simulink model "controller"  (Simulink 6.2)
settings: Solver=ode45  StartTime=0.0  StopTime=10.0  RelTol=1e-3
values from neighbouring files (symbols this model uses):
  calfa = cos(alfa0*d2r)    [run.m]
  d2r = pi/180    (= 0.0174532925199)    [run.m]
  Kfilt = (wd1^2*wd2^2*wd3^2*wd4^2*wd5^2*wd6^2)/(wn1^2*wn2^2*wn3^2*wn4^2*wn5^2*wn6^2)    (= 0.818930549142)    [run.m]
  klr = lqr(Ap4,Bp4,Q,R)    [run.m]
  kls = lqr(Ap3,Bp3,Q,R)    [run.m]
  salfa = sin(alfa0*d2r)    [run.m]
  Thet0 = 40    [run.m]
  V0 = 18640    [run.m]
  wd1 = 29    [run.m]
  wd2 = 37    [run.m]
  wd3 = 40    [run.m]
  wd4 = 48    [run.m]
  wd5 = 63    [run.m]
  wd6 = 68    [run.m]
  wd7 = 34    [run.m]
  wd8 = 19.1    [run.m]
  wlp = 6.6    [run.m]
  wlp2 = 12    [run.m]
  wlpr = 12    [run.m]
  wn1 = 30    [run.m]
  wn2 = 37.9    [run.m]
  wn3 = 40.2    [run.m]
  wn4 = 48.6    [run.m]
  wn5 = 64    [run.m]
  wn6 = 68.6    [run.m]
  wn7 = 34    [run.m]
  wn8 = 19.1    [run.m]
  zd1 = 0.12    [run.m]
  zd2 = 0.12    [run.m]
  zd3 = 0.1    [run.m]
  zd4 = 0.1    [run.m]
  zd5 = 0.1    [run.m]
  zd6 = 0.1    [run.m]
  zd7 = 0.1    [run.m]
  zd8 = 0.1    [run.m]
  zlp = 0.9    [run.m]
  zlp2 = 0.7    [run.m]
  zlpr = 0.7    [run.m]
  zn1 = 0.008    [run.m]
  zn2 = 0.01    [run.m]
  zn3 = 0.01    [run.m]
  zn4 = 0.02    [run.m]
  zn5 = 0.01    [run.m]
  zn6 = 0.01    [run.m]
  zn7 = 0.01    [run.m]
  zn8 = 0.01    [run.m]

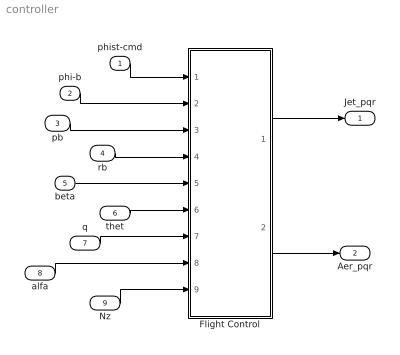
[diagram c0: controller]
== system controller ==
  phist-cmd : Inport  Port=1  LatchInput=off
  phi-b : Inport  Port=2  LatchInput=off
  pb : Inport  Port=3  LatchInput=off
  rb : Inport  Port=4  LatchInput=off
  beta : Inport  Port=5  LatchInput=off
  thet : Inport  Port=6  LatchInput=off
  q : Inport  Port=7  LatchInput=off
  alfa : Inport  Port=8  LatchInput=off
  Nz : Inport  Port=9  LatchInput=off
  Flight Control : Subsystem
  Jet_pqr : Outport
  Aer_pqr : Outport  Port=2
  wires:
  Flight Control/1(Jet_pqr) -> Jet_pqr/1
  Flight Control/2(Aer_pqr) -> Aer_pqr/1
  phi-b/1 -> Flight Control/2(phi)
  pb/1 -> Flight Control/3(pb)
  rb/1 -> Flight Control/4(rb)
  beta/1 -> Flight Control/5(beta)
  thet/1 -> Flight Control/6(thet)
  q/1 -> Flight Control/7(q)
  alfa/1 -> Flight Control/8(alfa)
  Nz/1 -> Flight Control/9(Nz)
  phist-cmd/1 -> Flight Control/1(phis-cmd)

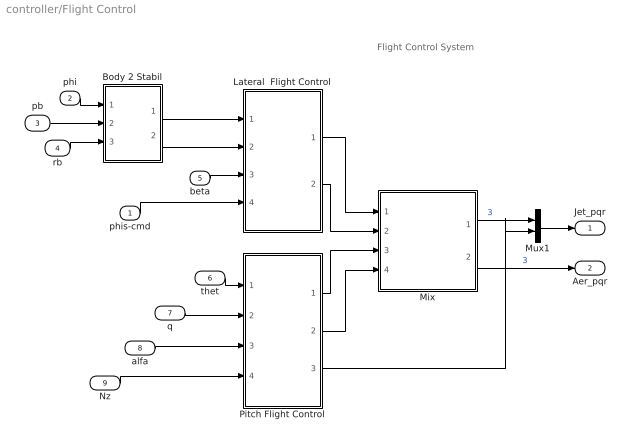
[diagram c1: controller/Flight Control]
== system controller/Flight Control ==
  note: Flight Control System
  phis-cmd : Inport  Port=1  LatchInput=off
  phi : Inport  Port=2  LatchInput=off
  pb : Inport  Port=3  LatchInput=off
  rb : Inport  Port=4  LatchInput=off
  beta : Inport  Port=5  LatchInput=off
  thet : Inport  Port=6  LatchInput=off
  q : Inport  Port=7  LatchInput=off
  alfa : Inport  Port=8  LatchInput=off
  Nz : Inport  Port=9  LatchInput=off
  Body 2 Stabil : Subsystem
  Lateral  Flight Control : Subsystem
  Mix : Subsystem
  Mux1 : Mux  Inputs=[3,1]
  Pitch Flight Control : Subsystem
  Jet_pqr : Outport
  Aer_pqr : Outport  Port=2
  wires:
  Lateral  Flight Control/1(rcs_PR) -> Mix/1(Rcs_PR)
  Lateral  Flight Control/2(aero_PR) -> Mix/2(Aer_PR)
  Pitch Flight Control/1(rcs_Q) -> Mix/3(Rcs_Q)
  Pitch Flight Control/2(aero_Q) -> Mix/4(Aer_Q)
  beta/1 -> Lateral  Flight Control/3(beta)
  Mix/2(Aer_pqr) -> Aer_pqr/1  "3"
  thet/1 -> Pitch Flight Control/1(thet)
  q/1 -> Pitch Flight Control/2(q)
  alfa/1 -> Pitch Flight Control/3(alf)
  Body 2 Stabil/2(r_s) -> Lateral  Flight Control/2(rs)
  Body 2 Stabil/1(p_s) -> Lateral  Flight Control/1(ps)
  rb/1 -> Body 2 Stabil/3(r_b)
  pb/1 -> Body 2 Stabil/2(p_b)
  phi/1 -> Body 2 Stabil/1(phi)
  Nz/1 -> Pitch Flight Control/4(Nz)
  Mix/1(Jet_pqr) -> Mux1/1  "3"
  Pitch Flight Control/3(Nzfb) -> Mux1/2
  Mux1/1 -> Jet_pqr/1
  phis-cmd/1 -> Lateral  Flight Control/4(phi-cmd)

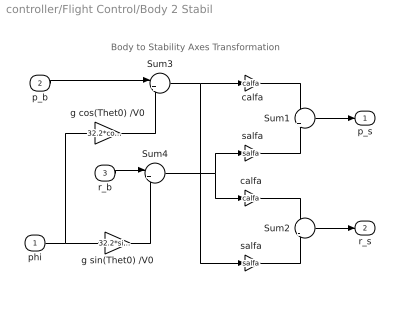
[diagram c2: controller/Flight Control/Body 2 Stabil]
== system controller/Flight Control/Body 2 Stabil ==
  note: Body to Stability Axes Transformation
  phi : Inport  Port=1  LatchInput=off
  p_b : Inport  Port=2  LatchInput=off
  r_b : Inport  Port=3  LatchInput=off
  Sum1 : Sum  Inputs=+|+
  Sum2 : Sum  Inputs=+|-
  Sum3 : Sum  Inputs=|++
  Sum4 : Sum  Inputs=|+-
  calfa : Gain  Gain=calfa
  "calfa " : Gain  Gain=calfa
  g cos(Thet0) /V0 : Gain  Gain=32.2*cos(Thet0*d2r)/V0
  g sin(Thet0) /V0 : Gain  Gain=32.2*sin(Thet0*d2r)/V0
  salfa : Gain  Gain=salfa
  "salfa " : Gain  Gain=salfa
  p_s : Outport
  r_s : Outport  Port=2
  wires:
  Sum1/1 -> p_s/1
  Sum2/1 -> r_s/1
  p_b/1 -> Sum3/1
  r_b/1 -> Sum4/1
  g cos(Thet0) /V0/1 -> Sum3/2
  g sin(Thet0) /V0/1 -> Sum4/2
  phi/1 -> g cos(Thet0) /V0/1, g sin(Thet0) /V0/1
  Sum4/1 -> "calfa "/1, salfa/1
  Sum3/1 -> "salfa "/1, calfa/1
  calfa/1 -> Sum1/1
  salfa/1 -> Sum1/2
  "calfa "/1 -> Sum2/1
  "salfa "/1 -> Sum2/2

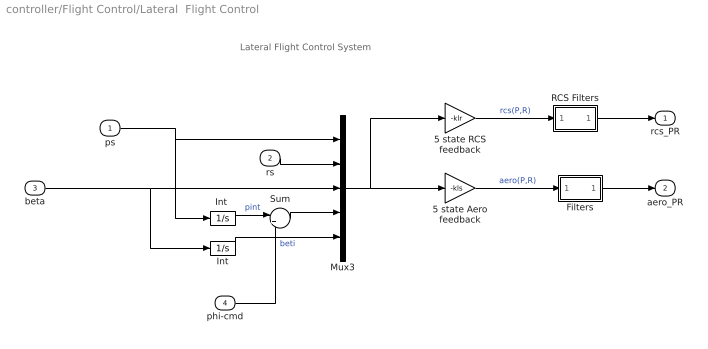
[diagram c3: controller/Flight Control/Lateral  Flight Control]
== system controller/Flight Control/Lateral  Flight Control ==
  note: Lateral Flight Control System
  ps : Inport  Port=1  LatchInput=off
  rs : Inport  Port=2  LatchInput=off
  beta : Inport  Port=3  LatchInput=off
  phi-cmd : Inport  Port=4  LatchInput=off
  5 state Aero feedback : Gain  Gain=-kls  Multiplication=Matrix(K*u)
  5 state RCS feedback : Gain  Gain=-klr  Multiplication=Matrix(K*u)
  Filters : Subsystem
  Int : Integrator
  "Int " : Integrator
  Mux3 : Mux  Inputs=5
  RCS Filters : Subsystem
  Sum : Sum  Inputs=|+-
  rcs_PR : Outport
  aero_PR : Outport  Port=2
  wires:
  Int/1 -> Mux3/5  "beti"
  beta/1 -> Int/1, Mux3/3
  ps/1 -> "Int "/1, Mux3/1
  Mux3/1 -> 5 state Aero feedback/1, 5 state RCS feedback/1
  rs/1 -> Mux3/2
  5 state RCS feedback/1 -> RCS Filters/1(In)  "rcs(P,R)"
  5 state Aero feedback/1 -> Filters/1(In)  "aero(P,R)"
  Filters/1(Ou) -> aero_PR/1
  RCS Filters/1(Ou) -> rcs_PR/1
  "Int "/1 -> Sum/1  "pint"
  Sum/1 -> Mux3/4
  phi-cmd/1 -> Sum/2

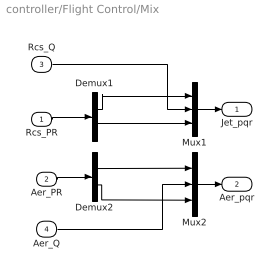
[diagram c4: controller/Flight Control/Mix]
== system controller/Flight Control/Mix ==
  Rcs_PR : Inport  Port=1  LatchInput=off
  Aer_PR : Inport  Port=2  LatchInput=off
  Rcs_Q : Inport  Port=3  LatchInput=off
  Aer_Q : Inport  Port=4  LatchInput=off
  Demux1 : Demux  Outputs=2
  Demux2 : Demux  Outputs=2
  Mux1 : Mux  Inputs=3
  Mux2 : Mux  Inputs=3
  Jet_pqr : Outport
  Aer_pqr : Outport  Port=2
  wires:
  Demux1/1 -> Mux1/1
  Demux1/2 -> Mux1/3
  Demux2/1 -> Mux2/1
  Demux2/2 -> Mux2/3
  Mux1/1 -> Jet_pqr/1
  Rcs_PR/1 -> Demux1/1
  Aer_PR/1 -> Demux2/1
  Aer_Q/1 -> Mux2/2
  Mux2/1 -> Aer_pqr/1
  Rcs_Q/1 -> Mux1/2

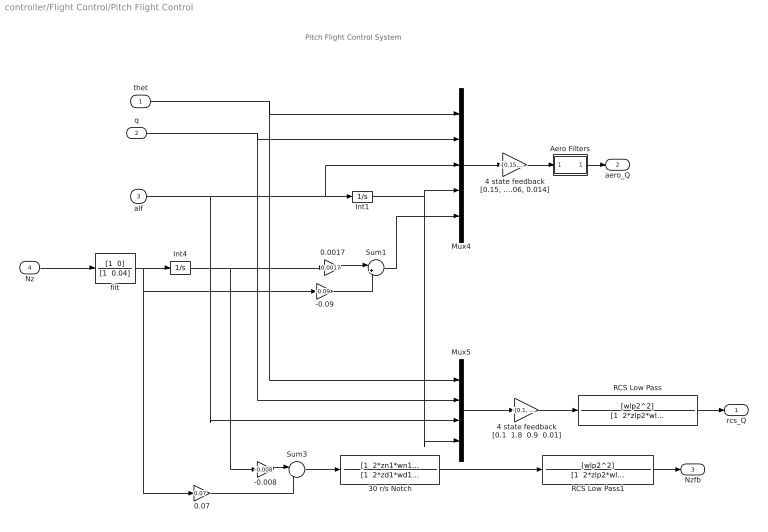
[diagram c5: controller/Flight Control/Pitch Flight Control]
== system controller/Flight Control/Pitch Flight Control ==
  note: Pitch Flight Control System
  thet : Inport  Port=1  LatchInput=off
  q : Inport  Port=2  LatchInput=off
  alf : Inport  Port=3  LatchInput=off
  Nz : Inport  Port=4  LatchInput=off
  -0.008 : Gain  Gain=-0.008
  -0.09 : Gain  Gain=-0.09
  0.0017 : Gain  Gain=0.0017
  0.07 : Gain  Gain=0.07
  30 r/s Notch : TransferFcn  Numerator="[1  2*zn1*wn1  wn1^2]"  Denominator="[1  2*zd1*wd1  wd1^2]"
  4 state feedback [0.1  1.8  0.9  0.01] : Gain  Gain="-[0.1,   1.8,   0.9,    0.01]"  Multiplication=Matrix(K*u)
  "4 state feedback [0.15, 2, 0.9, 0.06, 0.014]" : Gain  Gain="-[0.15,   2,   0.9,    0.06,   0.015]"  Multiplication=Matrix(K*u)
  Aero Filters : Subsystem
  Int1 : Integrator
  Int4 : Integrator
  Mux4 : Mux  Inputs=5
  Mux5 : Mux
  RCS Low Pass : TransferFcn  Numerator=[wlp2^2]  Denominator="[1  2*zlp2*wlp2  wlp2^2]"
  RCS Low Pass1 : TransferFcn  Numerator=[wlp2^2]  Denominator="[1  2*zlp2*wlp2  wlp2^2]"
  Sum1 : Sum  Inputs=|++
  Sum3 : Sum  Inputs=|++
  filt : TransferFcn  Numerator="[1  0]"  Denominator="[1  0.04]"
  rcs_Q : Outport
  aero_Q : Outport  Port=2
  Nzfb : Outport  Port=3
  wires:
  alf/1 -> Mux5/3, Mux4/3, Int1/1
  filt/1 -> 0.07/1, -0.09/1, Int4/1
  Int4/1 -> -0.008/1, 0.0017/1
  -0.008/1 -> Sum3/1
  0.07/1 -> Sum3/2
  4 state feedback [0.1  1.8  0.9  0.01]/1 -> RCS Low Pass/1
  Mux5/1 -> 4 state feedback [0.1  1.8  0.9  0.01]/1
  "4 state feedback [0.15, 2, 0.9, 0.06, 0.014]"/1 -> Aero Filters/1(in)
  Mux4/1 -> "4 state feedback [0.15, 2, 0.9, 0.06, 0.014]"/1
  Sum1/1 -> Mux4/5
  Nz/1 -> filt/1
  -0.09/1 -> Sum1/2
  0.0017/1 -> Sum1/1
  q/1 -> Mux5/2, Mux4/2
  thet/1 -> Mux5/1, Mux4/1
  Int1/1 -> Mux5/4, Mux4/4
  Sum3/1 -> 30 r/s Notch/1
  Aero Filters/1(ot) -> aero_Q/1
  RCS Low Pass/1 -> rcs_Q/1
  RCS Low Pass1/1 -> Nzfb/1
  30 r/s Notch/1 -> RCS Low Pass1/1

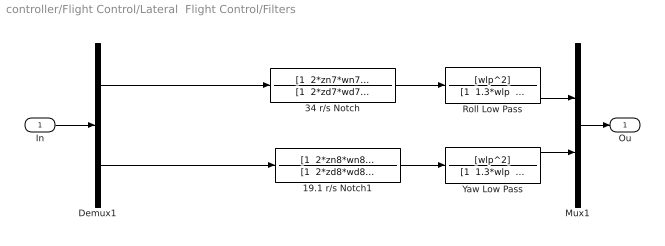
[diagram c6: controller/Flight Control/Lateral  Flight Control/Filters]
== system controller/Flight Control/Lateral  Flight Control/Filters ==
  In : Inport  Port=1  LatchInput=off
  19.1 r/s Notch1 : TransferFcn  Numerator="[1  2*zn8*wn8  wn8^2]"  Denominator="[1  2*zd8*wd8  wd8^2]"
  34 r/s Notch : TransferFcn  Numerator="[1  2*zn7*wn7  wn7^2]"  Denominator="[1  2*zd7*wd7  wd7^2]"
  Demux1 : Demux  Outputs=2
  Mux1 : Mux  Inputs=2
  Roll Low Pass : TransferFcn  Numerator=[wlp^2]  Denominator="[1  1.3*wlp  wlp^2]"
  Yaw Low Pass : TransferFcn  Numerator=[wlp^2]  Denominator="[1  1.3*wlp  wlp^2]"
  Ou : Outport
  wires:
  In/1 -> Demux1/1
  Demux1/1 -> 34 r/s Notch/1
  Mux1/1 -> Ou/1
  Roll Low Pass/1 -> Mux1/1
  Demux1/2 -> 19.1 r/s Notch1/1
  Yaw Low Pass/1 -> Mux1/2
  34 r/s Notch/1 -> Roll Low Pass/1
  19.1 r/s Notch1/1 -> Yaw Low Pass/1

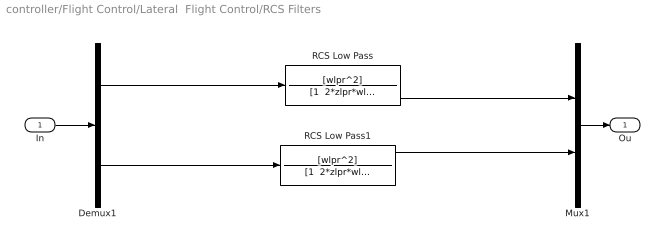
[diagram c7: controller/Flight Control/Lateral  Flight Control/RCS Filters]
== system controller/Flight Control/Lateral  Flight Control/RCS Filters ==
  In : Inport  Port=1  LatchInput=off
  Demux1 : Demux  Outputs=2
  Mux1 : Mux  Inputs=2
  RCS Low Pass : TransferFcn  Numerator=[wlpr^2]  Denominator="[1  2*zlpr*wlpr  wlpr^2]"
  RCS Low Pass1 : TransferFcn  Numerator=[wlpr^2]  Denominator="[1  2*zlpr*wlpr  wlpr^2]"
  Ou : Outport
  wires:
  In/1 -> Demux1/1
  Demux1/1 -> RCS Low Pass/1
  Mux1/1 -> Ou/1
  Demux1/2 -> RCS Low Pass1/1
  RCS Low Pass/1 -> Mux1/1
  RCS Low Pass1/1 -> Mux1/2

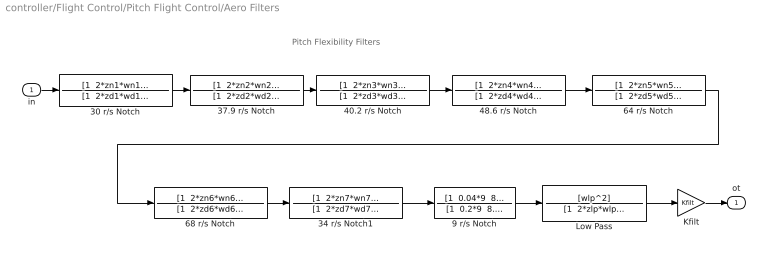
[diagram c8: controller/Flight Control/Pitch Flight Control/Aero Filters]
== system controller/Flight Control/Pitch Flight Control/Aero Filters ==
  note: Pitch Flexibility Filters
  in : Inport  Port=1  LatchInput=off
  30 r/s Notch : TransferFcn  Numerator="[1  2*zn1*wn1  wn1^2]"  Denominator="[1  2*zd1*wd1  wd1^2]"
  34 r/s Notch1 : TransferFcn  Numerator="[1  2*zn7*wn7  wn7^2]"  Denominator="[1  2*zd7*wd7  wd7^2]"
  37.9 r/s Notch : TransferFcn  Numerator="[1  2*zn2*wn2  wn2^2]"  Denominator="[1  2*zd2*wd2  wd2^2]"
  40.2 r/s Notch : TransferFcn  Numerator="[1  2*zn3*wn3  wn3^2]"  Denominator="[1  2*zd3*wd3  wd3^2]"
  48.6 r/s Notch : TransferFcn  Numerator="[1  2*zn4*wn4  wn4^2]"  Denominator="[1  2*zd4*wd4  wd4^2]"
  64 r/s Notch : TransferFcn  Numerator="[1  2*zn5*wn5  wn5^2]"  Denominator="[1  2*zd5*wd5  wd5^2]"
  68 r/s Notch : TransferFcn  Numerator="[1  2*zn6*wn6  wn6^2]"  Denominator="[1  2*zd6*wd6  wd6^2]"
  9 r/s Notch : TransferFcn  Numerator="[1  0.04*9  8.5^2]"  Denominator="[1  0.2*9  8.5^2]"
  Kfilt : Gain  Gain=Kfilt
  Low Pass : TransferFcn  Numerator=[wlp^2]  Denominator="[1  2*zlp*wlp  wlp^2]"
  ot : Outport
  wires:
  in/1 -> 30 r/s Notch/1
  30 r/s Notch/1 -> 37.9 r/s Notch/1
  37.9 r/s Notch/1 -> 40.2 r/s Notch/1
  40.2 r/s Notch/1 -> 48.6 r/s Notch/1
  Kfilt/1 -> ot/1
  68 r/s Notch/1 -> 34 r/s Notch1/1
  Low Pass/1 -> Kfilt/1
  48.6 r/s Notch/1 -> 64 r/s Notch/1
  64 r/s Notch/1 -> 68 r/s Notch/1
  9 r/s Notch/1 -> Low Pass/1
  34 r/s Notch1/1 -> 9 r/s Notch/1
